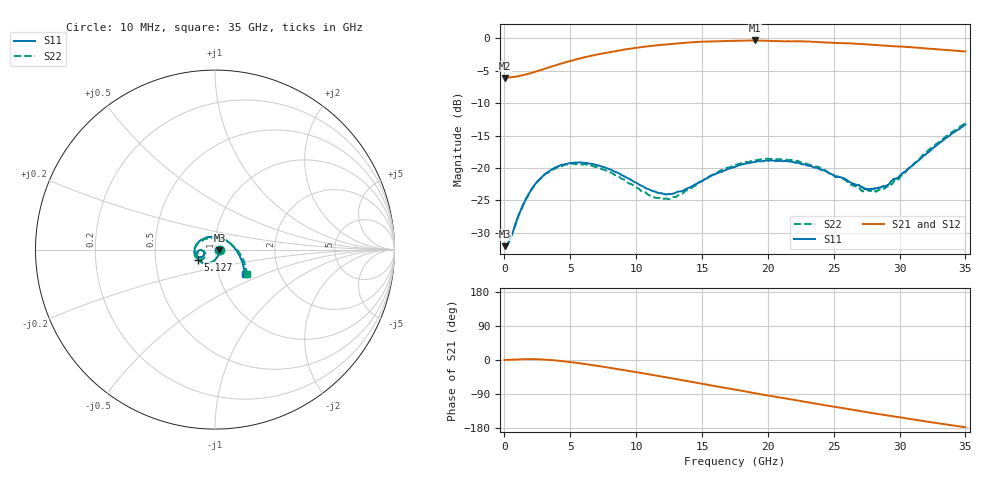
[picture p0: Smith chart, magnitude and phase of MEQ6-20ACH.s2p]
! MARKI MICROWAVE INC.
! Email:  support@markimicrowave.com  Phone:  408-778-4200
! Model Number:  MEQ6-20ACH  Date:  6/18
! Filename:		MEQ6-20ACH.S2P  Version: 1.0
! Description:  2-port S-parameter data for chip equalizer
! Features:		Low Insertion Loss, Excellent Return Loss
! Frequency Measured: 	10 MHz to 35 GHz
!S2P File: Measurements: S11, S21, S12, S22:
# Hz S  dB  R 50
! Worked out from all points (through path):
!   1601 points, 10 MHz to 35 GHz, reference 50 ohm
!   highest |S21| = -0.31 dB at 19.04 GHz (marker M1); lowest = -6.1 dB at 10 MHz (marker M2)
!   group delay of S21, straight-line fit = 15.7 ps
!   lowest |S11| = -32.1 dB at 53.74 MHz (marker M3), VSWR 1.05, Z = 52.5 - j0.39 ohm
!   |S11| at or under -10 dB: start of sweep to end of sweep
!   |S22| runs from -31.9 to -13.1 dB; largest |S21 - S12| = 0.0095
!   S11 on the Smith chart (normalised r, x): 10 MHz: 1.05, -0.01; 5.127 GHz: 0.82, -0.09; 35 GHz: 1.34, -0.39
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1e7  -32.01 -6.3  -6.10 0.1  -6.06 -0.0  -31.70 -8.1
5.37375e7  -32.06 -8.6  -6.08 0.2  -6.05 0.0  -31.76 -9.4
3.380312e8  -31.42 -29.9  -6.02 0.7  -6.02 0.6  -31.32 -30.5
1.518944e9  -25.21 -87.1  -5.62 2.4  -5.61 2.4  -25.21 -87.0
2.371825e9  -22.37 -107.7  -5.11 2.2  -5.12 2.2  -22.56 -107.6
3.596475e9  -20.22 -129.0  -4.32 -0.3  -4.32 -0.3  -20.25 -128.9
5.127288e9  -19.21 -149.2  -3.40 -6.0  -3.40 -6.0  -19.30 -148.8
5.848956e9  -19.15 -156.9  -3.02 -9.3  -3.02 -9.3  -19.46 -156.4
7.139212e9  -19.59 -168.0  -2.43 -15.8  -2.43 -15.9  -19.89 -167.4
8.910581e9  -21.09 -176.9  -1.77 -25.6  -1.77 -25.7  -21.67 -175.8
1.168791e10  -23.83 -170.5  -1.03 -42.2  -1.02 -42.1  -24.61 -164.3
1.304378e10  -23.77 -159.0  -0.78 -50.4  -0.77 -50.5  -24.42 -150.3
1.496822e10  -22.04 -150.8  -0.50 -62.5  -0.51 -62.4  -22.04 -141.7
1.7505e10  -19.79 -156.9  -0.36 -78.1  -0.36 -78.3  -19.55 -148.8
1.903581e10  -19.06 -166.1  -0.31 -87.7  -0.32 -87.6  -18.83 -157.7
2.183501e10  -19.03 172.5  -0.45 -104.3  -0.47 -104.6  -18.76 -179.3
2.334396e10  -19.75 158.1  -0.51 -113.5  -0.50 -113.3  -19.61 166.4
2.518093e10  -21.39 135.4  -0.69 -124.2  -0.66 -124.6  -21.27 144.5
2.721472e10  -22.98 96.1  -0.87 -136.0  -0.87 -135.7  -23.61 103.8
2.918291e10  -22.50 46.5  -1.15 -146.7  -1.13 -147.1  -22.74 50.8
3.152287e10  -18.69 0.1  -1.44 -159.6  -1.47 -159.4  -18.57 0.5
3.5e10  -13.27 -39.5  -2.00 -177.3  -1.99 -177.2  -13.09 -37.2
